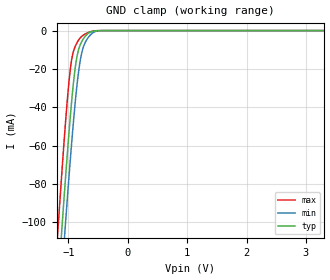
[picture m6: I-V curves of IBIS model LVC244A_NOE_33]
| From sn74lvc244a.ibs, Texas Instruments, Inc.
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[Model]   LVC244A_NOE_33
Model_type  Input
Vinl=0.8
Vinh=2.0
| variable   typ   min   max
C_comp   2.51pF   1.98pF   3.27pF
[Temperature Range]   40   100   -40
| Ambient temperature   25   85   -40
[Voltage range]   3.3   3   3.6
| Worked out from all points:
|   GND clamp passes 1 mA (typ) near -0.64 V on its own axis
[GND Clamp]
| LVC244A_NOE_33
|   Voltage   I(typ)   I(min)   I(max)
-5.5V     -2.303A    -2.296A    -2.31A
-1.185V   -137.1mA   -160.4mA   -108mA
-1.12V    -107.8mA   -131.4mA   -78.37mA
-1.105V   -101.2mA   -124.8mA   -71.74mA
-1.07V    -85.97mA   -109.6mA   -56.7mA
-1.055V   -79.59mA   -103.1mA   -50.5mA
-960mV    -42.03mA   -64.28mA   -18.31mA
-860mV    -14.34mA   -29.75mA   -6.633mA
-805mV    -7.737mA   -16.48mA   -3.993mA
-755mV    -4.658mA   -9.303mA   -2.51mA
-600mV    -473uA     -1.442mA   -357.6uA
3.3V      76.2pA     213.1pA    43.07pA
